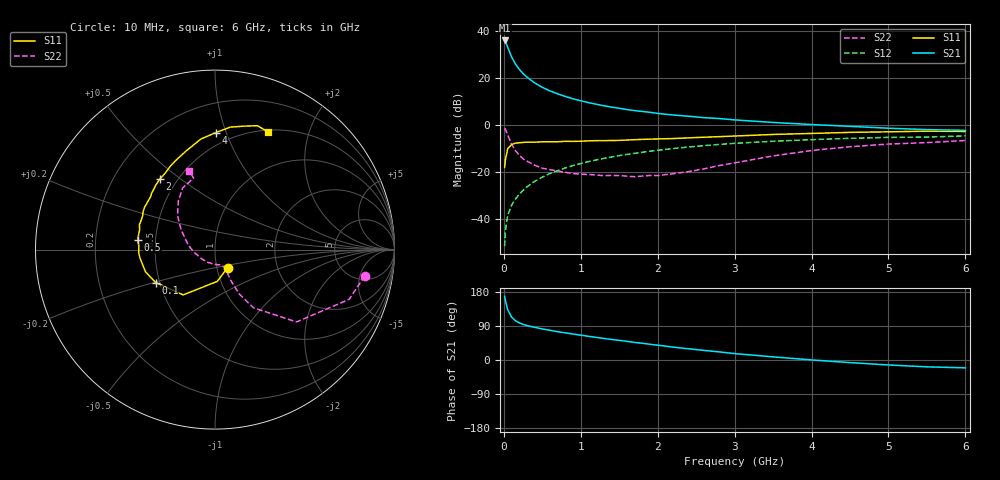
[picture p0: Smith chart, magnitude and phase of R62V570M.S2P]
! SIEMENS Small Signal Semiconductors
! BFR193
! Si NPN RF Bipolar Junction Transistor in SOT23
! VCE = 2.5 V  IC = 70 mA
! Common Emitter S-Parameters:  May  1996
# GHz  S  MA  R  50
!  f  S11  S21  S12  S22
! GHz  MAG  ANG  MAG  ANG  MAG  ANG  MAG  ANG
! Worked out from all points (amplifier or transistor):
!   36 points, 10 MHz to 6 GHz, reference 50 ohm
!   highest |S21| = 35.9 dB at 10 MHz (marker M1)
!   |S21| within 3 dB of that: start of sweep to 51.73 MHz
!   unconditionally stable (mu >= 1): 267.4 MHz to 2.104 GHz
!   at 250 MHz: K = 1.00, MSG = 24.8 dB, |S12| = -27.9 dB
!   at 1.4 GHz: K = 1.03, MAG = 9.6 dB, |S12| = -13.7 dB
!   at 6 GHz: K = 0.97, MSG = 1.2 dB, |S12| = -4.8 dB
!   S11 on the Smith chart (normalised r, x): 10 MHz: 1.12, -0.23; 100 MHz: 0.47, -0.20; 500 MHz: 0.40, +0.05; 2 GHz: 0.40, +0.42; 4 GHz: 0.41, +0.92; 6 GHz: 0.52, +1.42
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0.01  0.1229 -55.4  62.21 168.0  0.0026 77.9  0.8475 -9.9
0.02  0.1774 -85.8  59.04 156.9  0.0055 79.9  0.7975 -20.3
0.05  0.3084 -125.1  44.76 132.9  0.0118 70.5  0.6072 -41.6
0.1  0.3782 -151.0  28 113.5  0.0192 69.8  0.388 -56.6
0.15  0.4066 -162.3  19.8 103.7  0.0261 71.7  0.2823 -61.3
0.2  0.4124 -168.7  15.19 98.1  0.0332 74.2  0.2251 -62.3
0.25  0.4207 -173.6  12.25 94.0  0.0403 75.2  0.1877 -62.9
0.3  0.4252 -177.5  10.29 90.9  0.0477 76.0  0.1679 -62.6
0.4  0.425 177.0  7.793 86.4  0.0622 76.1  0.1378 -61.7
0.5  0.4337 173.2  6.253 82.0  0.0767 75.2  0.1187 -61.5
0.6  0.4339 168.8  5.25 78.4  0.0915 74.3  0.1105 -62.8
0.7  0.4344 165.2  4.548 74.6  0.1057 73.4  0.1036 -64.6
0.9  0.4424 158.8  3.559 68.5  0.1354 70.7  0.0913 -69.1
1.1  0.4535 152.0  2.959 62.5  0.164 68.0  0.0873 -76.7
1.4  0.4616 143.0  2.369 54.2  0.2057 63.4  0.0835 -89.3
2  0.499 128.0  1.742 39.2  0.2856 53.9  0.0827 -131.3
2.2  0.5081 123.2  1.611 34.0  0.3111 50.8  0.0906 -144.5
3.5  0.6211 97.3  1.118 8.3  0.4448 29.4  0.2169 150.0
4  0.6524 89.5  1.01 0.2  0.4817 22.3  0.2824 137.7
4.5  0.6878 82.9  0.924 -6.9  0.5138 15.1  0.3401 126.9
5.5  0.73 71.0  0.787 -18.1  0.5459 1.4  0.4167 106.6
6  0.7186 65.7  0.76 -20.7  0.5786 -2.6  0.4606 108.3
